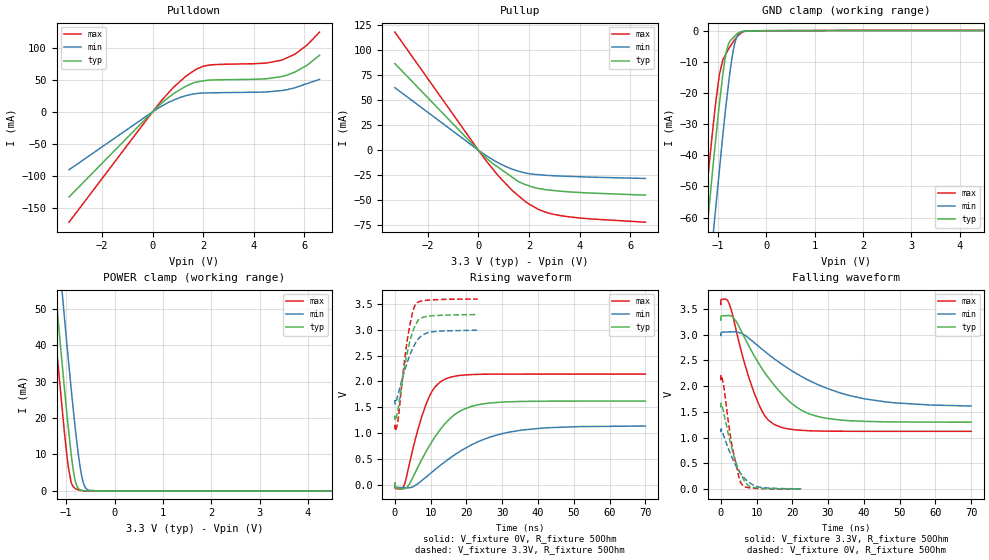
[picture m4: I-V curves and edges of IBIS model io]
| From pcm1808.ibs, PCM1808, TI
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|   io Model
[Model]   io
Model_type   I/O
Polarity   Non-Inverting
Enable   Active-Low
Vinl = 0.8
Vinh = 2
Vmeas = 1.65
Vref = 1.65
Cref = 20pF
Rref = 50
|   typ   min   max
|   (nom PVT)   (fast PVT)   (slow PVT)
C_comp   1.540e-12   1.477e-12   1.631e-12
|ON state : BUFFER OUTPUT TURNED HIGH
|C_comp   1.684e-12   1.608e-12   1.755e-12
|OFF state: BUFFER IN HIGH IMPEDANCE
|C_comp   1.397e-12   1.346e-12   1.508e-12
| Where nom  PVT is Nominal Process, 3.3V, 27C
|   Fast PVT is Strong Process,  3.6V, -40C
|   Slow PVT is Weak Process,   3V, 125C
[Voltage Range]   3.3   3   3.6
|Ambient Temperature   25   85   -40
|Junction Temperature
[Temperature Range]   27   125   -40
[Pullup Reference]   3.3   3   3.6
[Pulldown Reference]   0   0   0
[Power Clamp Reference]   3.3   3   3.6
[GND Clamp Reference]   0   0   0
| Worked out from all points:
|   slope of the pulldown table from 0 to 0.495 V, typ, clamps not added: 27.1 ohm
|   slope of the pullup table from 0 to 0.495 V, typ, clamps not added: 41.6 ohm
|   GND clamp passes 1 mA (typ) near -0.60 V on its own axis
|   POWER clamp passes 1 mA (typ) near -0.76 V on its own axis
|   falling waveform, V_fixture 3.3V, R_fixture 50Ohm: 20-80 % time 12.3ns typ, 21ns min, 6.6ns max; typ from 3.3 V to 1.3 V
|   rising waveform, V_fixture 0V, R_fixture 50Ohm: 20-80 % time 9.31ns typ, 16ns min, 5.53ns max; typ from 0 V to 1.62 V
|   rising waveform, V_fixture 3.3V, R_fixture 50Ohm: 20-80 % time 3.27ns typ, 4.14ns min, 2.77ns max; typ from 1.3 V to 3.3 V
|   falling waveform, V_fixture 0V, R_fixture 50Ohm: 20-80 % time 3.95ns typ, 4.88ns min, 3.06ns max; typ from 1.62 V to 0.003 V
[Pulldown]
|   Voltage   I(typ)   I(min)   I(max)
-3.3V     -133.4mA   -90.72mA   -172.9mA
327.6mV   12.54mA    8.343mA    16.53mA
831.6mV   28.63mA    18.43mA    38.64mA
1.307V    40.04mA    25.21mA    55.48mA
1.709V    46.6mA     28.52mA    66.3mA
2.023V    48.66mA    29.59mA    71.81mA
2.477V    50.09mA    29.97mA    74.11mA
4.471V    51.8mA     31.16mA    76.39mA
5.112V    55.45mA    33.43mA    81.12mA
5.648V    62.91mA    38.1mA     90.94mA
6.116V    73.42mA    44.41mA    105mA
6.6V      88.67mA    50.94mA    125mA
[GND Clamp]
|   Voltage   I(typ)   I(min)   I(max)
-3.3V     -425.4mA   -446.4mA   -412.3mA
-1.35V    -84.68mA   -106.9mA   -70.77mA
-1.284V   -73.45mA   -95.86mA   -59.97mA
-1.177V   -55.99mA   -78.08mA   -42.61mA
-1.109V   -44.79mA   -67.12mA   -32.18mA
-1.051V   -35.93mA   -57.97mA   -23.96mA
-968.4mV  -23.55mA   -44.81mA   -14.07mA
-821.7mV  -6.578mA   -22.64mA   -7.11mA
-729mV    -2.95mA    -10.93mA   -4.664mA
-648mV    -1.696mA   -3.876mA   -2.815mA
-513mV    -341.7uA   -301.8uA   -640.5uA
6.6V      65.17uA    30.87uA    124.2uA
[Pullup]
|   Voltage   I(typ)   I(min)   I(max)
-3.3V     86.28mA    62.29mA    117.7mA
327.6mV   -8.113mA   -5.747mA   -11.25mA
788.4mV   -17.13mA   -12.63mA   -25.59mA
1.332V    -26.84mA   -18.84mA   -40.05mA
1.558V    -30.87mA   -20.77mA   -44.87mA
1.818V    -33.93mA   -22.5mA    -50.44mA
2.477V    -38.59mA   -24.64mA   -60.13mA
2.826V    -39.79mA   -25.27mA   -63.06mA
3.244V    -40.9mA    -25.77mA   -65.21mA
4.471V    -42.77mA   -26.88mA   -68.54mA
6.6V      -44.8mA    -28.2mA    -71.76mA
[POWER Clamp]
|   Voltage   I(typ)   I(min)   I(max)
-3.3V     383.3mA    401.4mA    372mA
-1.29V    65.4mA     85.28mA    53mA
-1.17V    47.45mA    67.1mA     34.83mA
-1.112V   38.83mA    58.6mA     26.66mA
-1.04V    28.74mA    48.12mA    16.53mA
-957.6mV  17.61mA    36.36mA    6.693mA
-896.4mV  10.01mA    27.9mA     2.267mA
-818.4mV  3.042mA    17.89mA    731.3uA
-738mV    520.7uA    8.928mA    235.7uA
-660mV    87.45uA    2.93mA     77.59uA
-540mV    35.88uA    208.1uA    2.36uA
6.6V      0A         0A         0A
[Ramp]
R_load = 50
|   typ   min   max
dV/dt_r   0.970788/9.31475e-09   0.680717/1.59464e-08   1.2856/5.5277e-09
dV/dt_f   1.19833/1.22806e-08   0.830666/2.08912e-08   1.48476/6.59417e-09
[Falling Waveform]
V_fixture = 3.3V
V_fixture_min = 3V
V_fixture_max = 3.6V
R_fixture = 50Ohm
|   Time   V(typ)   V(min)   V(max)
0s        3.299V     2.999V     3.598V
2.288ns   3.371V     3.053V     3.61V
4.348ns   3.253V     3.052V     3.073V
9.272ns   2.599V     2.849V     1.883V
12.09ns   2.283V     2.686V     1.449V
14.76ns   2.034V     2.541V     1.264V
21.34ns   1.584V     2.237V     1.149V
27.98ns   1.397V     2.005V     1.128V
46.67ns   1.307V     1.69V      1.123V
70ns      1.301V     1.615V     1.123V
[Rising Waveform]
V_fixture = 0V
V_fixture_min = 0V
V_fixture_max = 0V
R_fixture = 50Ohm
|   Time   V(typ)   V(min)   V(max)
0s        0V         0V         0V
140ps     -64.3mV    -49.02mV   -78.64mV
2.46ns    -84.98mV   -63.47mV   -34.01mV
6.384ns   330.1mV    14.91mV    1.053V
8.88ns    660.1mV    153.9mV    1.588V
11.23ns   926.8mV    289.8mV    1.894V
14.25ns   1.197V     454.3mV    2.051V
21.34ns   1.515V     767.4mV    2.132V
31.84ns   1.605V     1.014V     2.142V
70ns      1.618V     1.135V     2.143V
[Rising Waveform]
V_fixture = 3.3V
V_fixture_min = 3V
V_fixture_max = 3.6V
R_fixture = 50Ohm
|   Time   V(typ)   V(min)   V(max)
0s        1.301V     1.603V     1.123V
184ps     1.252V     1.57V      1.054V
916ps     1.478V     1.753V     1.267V
2.428ns   2.164V     2.143V     2.251V
3.708ns   2.638V     2.421V     2.907V
4.932ns   2.957V     2.634V     3.331V
5.772ns   3.096V     2.745V     3.497V
6.84ns    3.206V     2.849V     3.549V
9.376ns   3.266V     2.951V     3.577V
23.16ns   3.297V     2.993V     3.598V
[Falling Waveform]
V_fixture = 0V
V_fixture_min = 0V
V_fixture_max = 0V
R_fixture = 50Ohm
|   Time   V(typ)   V(min)   V(max)
0s        1.618V     1.136V     2.143V
140ps     1.666V     1.167V     2.214V
916ps     1.461V     1.022V     1.964V
2.528ns   948.8mV    718.5mV    1.112V
3.452ns   700.3mV    570.2mV    738.8mV
5.056ns   375.2mV    358.8mV    242.9mV
5.992ns   244mV      264.3mV    85.03mV
8.42ns    45.38mV    110mV      24.61mV
11.96ns   17.04mV    28.81mV    9.951mV
22.53ns   3.099mV    7.137mV    746uV
